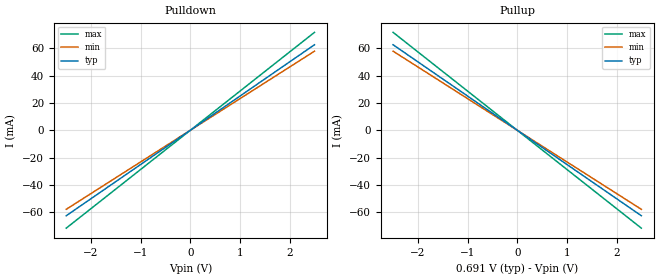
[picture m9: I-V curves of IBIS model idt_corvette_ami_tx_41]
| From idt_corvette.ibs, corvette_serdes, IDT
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|   model   idt_corvette_ami_tx_41
[Model] idt_corvette_ami_tx_41
Model_type Output
C_comp 400f 400f 400f
Cref = 0
[Model Spec]
Vmeas 0. 0. 0.
Vref 0. 0. 0.
[Temperature Range]  25 100 0
[Voltage Range] .691 .681 .584
[Algorithmic Model]
Executable Windows_VisualStudio5_32 idt_corvette_tx.dll   idt_corvette_tx.ami
Executable Windows_ver_64   idt_corvette_tx_64.dll   idt_corvette_tx.ami
Executable Linux_gcc4.1.2_32   idt_corvette_tx.linux.so   idt_corvette_tx.ami
Executable Linux_gcc3.2.3_64   idt_corvette_tx_64.linux.so idt_corvette_tx.ami
[End Algorithmic Model]
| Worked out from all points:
|   slope of the pulldown table from 0 to 0.104 V, typ, clamps not added: 40 ohm
|   slope of the pullup table from 0 to 0.104 V, typ, clamps not added: 40 ohm
[Pulldown]
-2.5V     -62.5mA    -57.8mA    -71.57mA
0V        0A         0A         0A
2.5V      62.5mA     57.8mA     71.57mA
[Pullup]
-2.5V     62.5mA     57.8mA     71.57mA
0V        0A         0A         0A
2.5V      -62.5mA    -57.8mA    -71.57mA
[Ramp]
dV/dt_r .23/22.4p .219/24.22p .206/19.562p
dV/dt_f .23/22.4p .219/24.22p .206/19.562p
